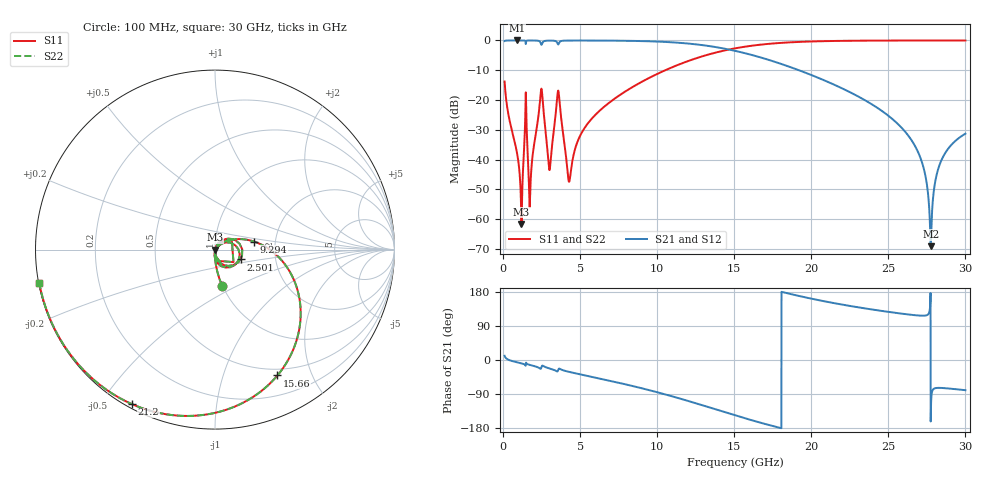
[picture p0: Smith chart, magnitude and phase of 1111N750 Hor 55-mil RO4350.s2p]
# GHz S MA R 50
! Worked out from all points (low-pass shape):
!   3201 points, 100 MHz to 30 GHz, reference 50 ohm
!   highest |S21| = -0.01 dB at 903.6 MHz (marker M1); lowest = -69.0 dB at 27.75 GHz (marker M2)
!   |S21| within 3 dB of the highest: start of sweep to 14.61 GHz
!   lowest |S11| = -61.6 dB at 1.193 GHz (marker M3), VSWR 1.00, Z = 50.1 - j0.033 ohm
!   |S11| at or under -10 dB: start of sweep to 10.52 GHz
!   |S22| runs from -61.6 to 0.0 dB; largest |S21 - S12| = 0
!   S11 on the Smith chart (normalised r, x): 100 MHz: 1.00, -0.42; 2.501 GHz: 1.32, -0.15; 9.294 GHz: 1.55, +0.15; 15.66 GHz: 0.42, -1.53; 21.2 GHz: 0.02, -0.60; 30 GHz: 0.00, -0.09
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0.1  0.2046 -78.9  0.9786 11.1  0.9786 11.1  0.2046 -78.9
0.9035625  0.01296 -93.7  0.9993 -6.0  0.9993 -6.0  0.01296 -93.7
1.193219  0.0008293 -23.4  0.9991 -8.9  0.9991 -8.9  0.0008293 -23.4
1.436156  0.04711 58.8  0.9843 -13.2  0.9843 -13.2  0.04711 58.8
1.781875  0.003985 54.1  0.9983 -13.4  0.9983 -13.4  0.003985 54.1
2.501344  0.1528 -21.2  0.8471 -18.0  0.8471 -18.0  0.1528 -21.2
3.005906  0.006684 -21.8  0.993 -22.2  0.993 -22.2  0.006684 -21.8
3.566531  0.1434 -17.0  0.8584 -27.7  0.8584 -27.7  0.1434 -17.0
4.276656  0.004248 -28.1  0.9953 -31.3  0.9953 -31.3  0.004248 -28.1
5.089563  0.02788 46.1  0.9964 -38.5  0.9964 -38.5  0.02788 46.1
9.29425  0.222 11.7  0.9712 -77.6  0.9712 -77.6  0.222 11.7
10.06978  0.2793 3.6  0.956 -85.8  0.956 -85.8  0.2793 3.6
15.05  0.7364 -56.3  0.6695 -145.9  0.6695 -145.9  0.7364 -56.3
15.65734  0.7828 -63.6  0.6147 -153.3  0.6147 -153.3  0.7828 -63.6
20.03956  0.9617 -108.8  0.2606 161.6  0.2606 161.6  0.9617 -108.8
21.19819  0.9773 -118.2  0.1953 152.2  0.1953 152.2  0.9773 -118.2
25.01978  0.9955 -143.8  0.05403 126.9  0.05403 126.9  0.9955 -143.8
26.99131  0.9969 -154.6  0.01229 117.3  0.01229 117.3  0.9969 -154.6
27.40244  0.997 -156.8  0.005411 117.3  0.005411 117.3  0.997 -156.8
27.74816  0.997 -158.5  0.0003528 -162.1  0.0003528 -162.1  0.997 -158.5
28.41156  0.997 -161.8  0.009329 -73.6  0.009329 -73.6  0.997 -161.8
30  0.9966 -169.3  0.02724 -79.7  0.02724 -79.7  0.9966 -169.3
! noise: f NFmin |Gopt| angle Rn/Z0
0.1  0.0006543  0.7306  1.341  0.0004839
3.417  0.03874  0.8375  25.08  0.04805
6.743  0.01757  0.4592  46.68  0.004719
10.06  0.02479  0.4584  64.1  0.005819
13.39  0.03652  0.5287  79.77  0.008564
16.7  0.05808  0.6494  96.67  0.0147
20.03  0.1064  0.7883  115.8  0.0303
23.35  0.2504  0.9044  135.1  0.08494
26.67  1.418  0.9821  153.1  0.994
30  0.9606  0.9729  169.2  0.07407
